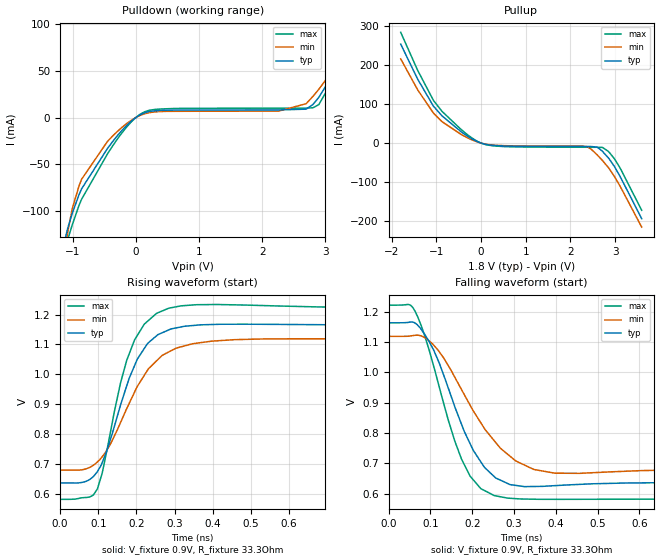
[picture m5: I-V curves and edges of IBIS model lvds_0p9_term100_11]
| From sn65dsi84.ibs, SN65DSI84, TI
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|   Model
[Model]   lvds_0p9_term100_11
Model_type   Output
Polarity   Non-Inverting
Vmeas = 0.9
Vref = 0.9
Cref = 1pF
Rref = 50
|   typ   min   max
C_comp   0.4797pF   0.3035pF   0.7186pF
[Voltage Range]   1.8   1.65   1.95
[Temperature Range]   27   125   -40
[Pullup Reference]   1.8   1.65   1.95
[Pulldown Reference]   -0   -0   -0
[Power Clamp Reference]   1.8   1.65   1.95
[GND Clamp Reference]   -0   -0   -0
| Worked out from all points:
|   slope of the pulldown table from 0 to 0.27 V, typ, clamps not added: 38.9 ohm
|   slope of the pullup table from 0 to 0.27 V, typ, clamps not added: 46.1 ohm
|   falling waveform, V_fixture 0.9V, R_fixture 33.3Ohm: 20-80 % time 90.4ps typ, 118ps min, 83.5ps max; typ from 1.16 V to 0.636 V
|   rising waveform, V_fixture 0.9V, R_fixture 33.3Ohm: 20-80 % time 84.4ps typ, 109ps min, 71.7ps max; typ from 0.636 V to 1.16 V
[Pulldown]
|   Voltage   I(typ)   I(min)   I(max)
-1.8V     -664mA     -698.6mA   -654.8mA
-1.103V   -124.3mA   -132.7mA   -135.5mA
-1.076V   -117.1mA   -120.7mA   -129.1mA
-1.006V   -101.7mA   -96.59mA   -113.9mA
-860.4mV  -75.94mA   -65.78mA   -87.08mA
-374.4mV  -26.17mA   -20.13mA   -30.86mA
-88.2mV   -4.784mA   -3.652mA   -5.748mA
144mV     5.141mA    4.062mA    6.208mA
2.261V    8.088mA    6.819mA    9.953mA
2.698V    8.927mA    14.76mA    10.02mA
2.898V    21.49mA    30.04mA    13.72mA
3.595V    96.25mA    93.35mA    94.7mA
[Pullup]
|   Voltage   I(typ)   I(min)   I(max)
-1.8V     253.9mA    216.1mA    284.3mA
-1.417V   163.3mA    136mA      185.8mA
-1.06V    93.72mA    76.1mA     108.5mA
-860.4mV  68.43mA    53.78mA    79.82mA
-261mV    14.71mA    11.16mA    17.75mA
3.6mV     -137.9uA   -109.5uA   -161.2uA
306mV     -6.217mA   -5.34mA    -7.253mA
2.369V    -8.748mA   -8.979mA   -10.64mA
2.596V    -10.35mA   -29.96mA   -10.71mA
2.876V    -42.02mA   -67.11mA   -24.82mA
3.109V    -85.23mA   -110.2mA   -63.62mA
3.595V    -194.2mA   -215.7mA   -172.5mA
[Ramp]
R_load = 33.3
|   typ   min   max
dV/dt_r   0.316806/8.43595e-11   0.263671/1.09262e-10   0.384007/7.17319e-11
dV/dt_f   0.316118/9.03588e-11   0.263526/1.18113e-10   0.38386/8.35145e-11
[Falling Waveform]
V_fixture = 0.9V
V_fixture_min = 0.9V
V_fixture_max = 0.9V
R_fixture = 33.3Ohm
C_fixture = 0F
|   Time   V(typ)   V(min)   V(max)
0s        1.163V     1.118V     1.221V
50ps      1.165V     1.119V     1.222V
63.2ps    1.162V     1.122V     1.201V
107.7ps   1.073V     1.089V     1.019V
174.4ps   828.1mV    942.5mV    713.3mV
220.5ps   704.5mV    833.2mV    616.1mV
252.7ps   655.8mV    773.9mV    593.2mV
303.8ps   626.8mV    707.7mV    583.2mV
397.5ps   626mV      667.1mV    580.9mV
1ns       636mV      679mV      581.4mV
[Rising Waveform]
V_fixture = 0.9V
V_fixture_min = 0.9V
V_fixture_max = 0.9V
R_fixture = 33.3Ohm
C_fixture = 0F
|   Time   V(typ)   V(min)   V(max)
0s        636.2mV    679.4mV    581.3mV
68ps      641.6mV    683.5mV    587.5mV
97.62ps   674mV      706.6mV    616.1mV
120.9ps   738.1mV    743mV      735.6mV
174.4ps   961.1mV    884.8mV    1.047V
202.4ps   1.051V     959.8mV    1.13V
252.7ps   1.129V     1.045V     1.204V
303.8ps   1.155V     1.088V     1.226V
397.5ps   1.167V     1.111V     1.234V
1ns       1.164V     1.119V     1.221V
